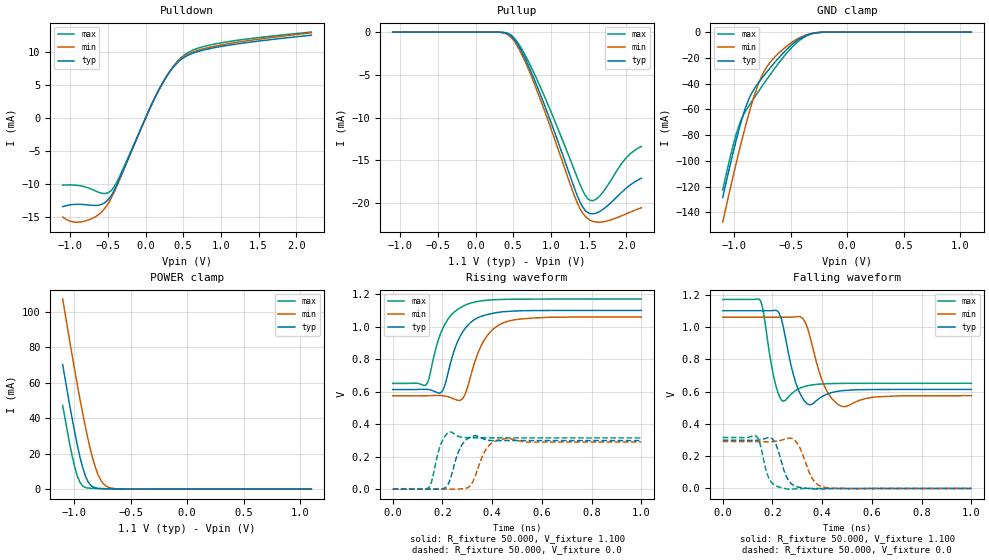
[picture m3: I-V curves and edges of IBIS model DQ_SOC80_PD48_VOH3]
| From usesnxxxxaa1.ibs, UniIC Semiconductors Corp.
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|   Model DQ_SOC80_PD48_VOH3
[Model] DQ_SOC80_PD48_VOH3
Model_type I/O
Polarity   Non-Inverting
Enable   Active-High
Vinl =  0.113V
Vinh =  0.253V
Vmeas =  0.183V
Rref =  50.000
Vref =  0.183V
C_comp   1.110pF   1.087pF   1.118pF
[Model Spec]
Vinh   0.253V   0.247V   0.265V
Vinl   0.113V   0.107V   0.125V
Vmeas   0.183V   NA   NA
Vref   0.183V   NA   NA
Rref   50.000   NA   NA
[Temperature Range]   25.000   0.125k   -40.000
[Voltage Range]   1.100V   1.060V   1.170V
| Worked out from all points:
|   slope of the pulldown table from 0 to 0.165 V, typ, clamps not added: 41.1 ohm
|   GND clamp passes 1 mA (typ) near -0.30 V on its own axis
|   POWER clamp passes 1 mA (typ) near -0.82 V on its own axis
|   rising waveform, R_fixture 50.000, V_fixture 1.100: 20-80 % time 76.5ps typ, 80.5ps min, 75.4ps max; typ from 0.613 V to 1.1 V
|   rising waveform, R_fixture 50.000, V_fixture 0.0: 20-80 % time 36.1ps typ, 44.8ps min, 28.9ps max; typ from 0 V to 0.299 V
|   falling waveform, R_fixture 50.000, V_fixture 1.100: 20-80 % time 39.8ps typ, 52.4ps min, 30.6ps max; typ from 1.1 V to 0.613 V
|   falling waveform, R_fixture 50.000, V_fixture 0.0: 20-80 % time 38.8ps typ, 46.4ps min, 31.7ps max; typ from 0.299 V to 0 V
[Pulldown]
|Voltage   I(typ)   I(min)   I(max)
-1.1V     -13.43mA   -15.01mA   -10.18mA
-930mV    -13.07mA   -15.78mA   -10.18mA
-726mV    -13.22mA   -15.3mA    -10.75mA
-556mV    -12.93mA   -13.9mA    -11.45mA
-454mV    -11.73mA   -12.11mA   -10.97mA
-352mV    -9.395mA   -9.553mA   -9.028mA
158mV     3.857mA    3.874mA    3.821mA
328mV     7.102mA    7.168mA    7.155mA
498mV     9.071mA    9.207mA    9.38mA
668mV     9.963mA    10.14mA    10.45mA
940mV     10.7mA     10.92mA    11.25mA
2.2V      12.53mA    12.89mA    13.01mA
[Pullup]
|Voltage   I(typ)   I(min)   I(max)
-1.1V     1nA        20.18nA    0A
432mV     -223uA     -332.2uA   -150.9uA
568mV     -1.57mA    -1.836mA   -1.333mA
738mV     -4.656mA   -5.117mA   -4.085mA
976mV     -9.963mA   -10.68mA   -8.789mA
1.316V    -18.32mA   -19.22mA   -16.24mA
1.418V    -20.39mA   -21.1mA    -18.43mA
1.486V    -21.07mA   -21.78mA   -19.43mA
1.554V    -21.24mA   -22.11mA   -19.69mA
1.622V    -21.08mA   -22.21mA   -19.37mA
1.996V    -18.26mA   -21.25mA   -14.72mA
2.2V      -17.08mA   -20.52mA   -13.36mA
[GND_clamp]
|Voltage   I(typ)   I(min)   I(max)
-1.1V     -128.5mA   -147.6mA   -122.6mA
-1.008V   -93.62mA   -112mA     -87.95mA
-962mV    -77.6mA    -95.05mA   -73.96mA
-893mV    -57.36mA   -71.21mA   -60.7mA
-847mV    -48.01mA   -56.81mA   -54.36mA
-801mV    -41.47mA   -44.23mA   -48.33mA
-755mV    -36.02mA   -34.19mA   -42.41mA
-709mV    -30.9mA    -26.94mA   -36.63mA
-525mV    -12.67mA   -10.3mA    -15.49mA
-387mV    -3.615mA   -3.065mA   -4.419mA
-249mV    -281uA     -330.6uA   -301.3uA
1.1V      0A         0A         0A
[POWER_clamp]
|Voltage   I(typ)   I(min)   I(max)
-1.1V     70.27mA    107.3mA    47.25mA
-1.039V   47.68mA    83.93mA    25.86mA
-993mV    31.88mA    66.94mA    12.35mA
-970mV    24.65mA    58.72mA    7.262mA
-947mV    18.06mA    50.74mA    3.761mA
-901mV    7.73mA     35.71mA    987.1uA
-855mV    2.348mA    22.46mA    514uA
-809mV    697.3uA    11.94mA    396.5uA
-763mV    321uA      5.097mA    322.7uA
-717mV    213.8uA    1.813mA    258.1uA
-556mV    65.24uA    79.15uA    81.64uA
1.1V      0A         0A         0A
[Ramp]
| variable   typ   min   max
dV/dt_r   0.179/36.360p   0.174/45.625p   0.189/29.256p
dV/dt_f   0.292/40.291p   0.291/52.891p   0.311/30.736p
R_load = 50.000
[Rising Waveform]
R_fixture= 50.000
V_fixture= 1.100
V_fixture_min= 1.060
V_fixture_max= 1.170
|time   V(typ)   V(min)   V(max)
0s        613mV      574.4mV    651mV
134ps     614.6mV    574.9mV    641.3mV
193ps     592.7mV    576.2mV    958.7mV
223ps     718.3mV    568.5mV    1.048V
272ps     942.7mV    547.1mV    1.116V
292ps     990.6mV    586.4mV    1.133V
311ps     1.023V     680.8mV    1.144V
366ps     1.069V     912.3mV    1.161V
446ps     1.092V     1.024V     1.168V
1ns       1.1V       1.06V      1.17V
[Rising Waveform]
R_fixture= 50.000
V_fixture= 0.0
V_fixture_min= 0.0
V_fixture_max= 0.0
|time   V(typ)   V(min)   V(max)
0s        1.965uV    15.9uV     367.9nV
148ps     122.4uV    -2.234uV   15.37mV
189ps     1.166mV    81.49uV    257.4mV
226ps     40.78mV    69.8uV     350.4mV
274ps     261.9mV    1.912mV    320.5mV
302ps     311.2mV    9.006mV    316.6mV
323ps     326.1mV    47.41mV    315.9mV
377ps     303.4mV    249mV      315.5mV
431ps     298.8mV    305mV      315.5mV
1ns       299.2mV    290.5mV    315.5mV
[Falling Waveform]
R_fixture= 50.000
V_fixture= 1.100
V_fixture_min= 1.060
V_fixture_max= 1.170
|time   V(typ)   V(min)   V(max)
0s        1.1V       1.06V      1.17V
152ps     1.1V       1.06V      1.161V
205ps     1.102V     1.06V      692.1mV
242ps     1.011V     1.06V      540.3mV
292ps     663.4mV    1.062V     604.6mV
322ps     556.9mV    1.053V     627.7mV
349ps     517.7mV    951.7mV    638.2mV
407ps     574.9mV    641.2mV    647.5mV
476ps     604.5mV    510.3mV    650.2mV
1ns       612.9mV    574.4mV    651mV
[Falling Waveform]
R_fixture= 50.000
V_fixture= 0.0
V_fixture_min= 0.0
V_fixture_max= 0.0
|time   V(typ)   V(min)   V(max)
0s        299.2mV    290.5mV    315.5mV
133ps     298.2mV    290.1mV    325.5mV
146ps     299.7mV    289.8mV    297.3mV
180ps     313.2mV    289.3mV    84.27mV
202ps     303.6mV    290.5mV    28.85mV
245ps     118.8mV    302.8mV    765.8uV
292ps     14.21mV    295.6mV    -2.332mV
357ps     -1.406mV   70.67mV    -162uV
407ps     -2.648mV   8.107mV    -13.75uV
1ns       4.281uV    19.63uV    2.011uV
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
